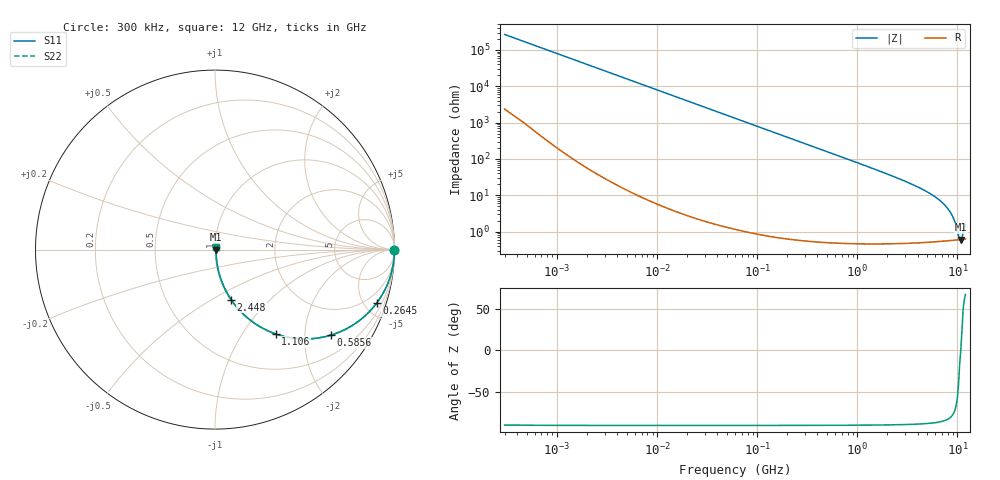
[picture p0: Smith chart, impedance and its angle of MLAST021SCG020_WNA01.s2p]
! MLAST021SCG020_WNA01  S-PARAMETER MODEL  ( General Type )
! Model Generated by TAIYO YUDEN Corporation (http://www.ty-top.com)
! Version 1.0
! TAIYO YUDEN Control No. 220901
! Copyright(c) 2022 TAIYO YUDEN CO.,LTD. All Rights Reserved.
! Product Description (link to TY-COMPAS)
! https://ds.yuden.co.jp/TYCOMPAS/or/detail?pn=MLAST021SCG020BWNA01&u=M
! Products Name : Multilayer Ceramic Capacitors
! Characteristics :
!  Capacitance : 2 pF , Rated Voltage : 25V , TCC : CG / C0G
!  Case Size : 0.25 x 0.125 / 0.0098 x 0.0049 [mm/inch] , Thickness : 0.125 / 0.0049 [mm/inch]
!  (Conditions: Temperature = 25 degC , DC Bias Current/Voltage = 0A / 0V)
! External Node Assignments :
!  1  o---| |---o  2
! GND o---------o GND
! Frequency Range : 0.3MHz  -  12000MHz  [ 401 STEP ]
# MHz S RI R 50
! Freq[MHz].  S11 Real  S11 Imag  S21 Real  S21 Imag  S12 Real  S12 Imag  S22 Real  S22 Imag
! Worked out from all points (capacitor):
!   401 points, 300 kHz to 12 GHz, reference 50 ohm
!   read as one part in series: C = 2 pF near 316.3 kHz
!   lowest |Z| = 606 mohm at 10.79 GHz (marker M1)
!   series resonance near 10.79 GHz, so ESL is about 110 pH
!   S11 on the Smith chart (normalised r, x): 300 kHz: open; 264.5 MHz: 1.01, -6.01; 585.6 MHz: 1.01, -2.71; 1.106 GHz: 1.01, -1.42; 2.448 GHz: 1.01, -0.62; 12 GHz: 1.01, +0.03
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0.3  1 -0.000377  3.48e-06 0.000377  3.48e-06 0.000377  1 -0.000377
1.769972  1 -0.00222  8.37e-06 0.00222  8.37e-06 0.00222  1 -0.00222
10.44266  0.9998 -0.0131  0.000182 0.0131  0.000182 0.0131  0.9998 -0.0131
60  0.9943 -0.075  0.00572 0.075  0.00572 0.075  0.9943 -0.075
129.3602  0.9741 -0.1583  0.0259 0.1583  0.0259 0.1583  0.9741 -0.1583
264.5085  0.8999 -0.2991  0.1001 0.2991  0.1001 0.2991  0.8999 -0.2991
353.9943  0.8339 -0.371  0.1661 0.371  0.1661 0.371  0.8339 -0.371
585.5907  0.6468 -0.4762  0.3532 0.4762  0.3532 0.4762  0.6468 -0.4762
804.7407  0.4916 -0.4975  0.5084 0.4975  0.5084 0.4975  0.4916 -0.4975
1105.905  0.3373 -0.4695  0.6627 0.4695  0.6627 0.4695  0.3373 -0.4695
2088.533  0.1214 -0.3203  0.8786 0.3203  0.8786 0.3203  0.1214 -0.3203
2448.343  0.09 -0.2787  0.91 0.2787  0.91 0.2787  0.09 -0.2787
4623.766  0.0238 -0.1354  0.9762 0.1354  0.9762 0.1354  0.0238 -0.1354
6879.757  0.0098 -0.066  0.9902 0.066  0.9902 0.066  0.0098 -0.066
7854.144  0.00763 -0.0452  0.9924 0.0452  0.9924 0.0452  0.00763 -0.0452
8732.115  0.00656 -0.029  0.9934 0.029  0.9934 0.029  0.00656 -0.029
9454.42  0.00612 -0.0171  0.9939 0.0171  0.9939 0.0171  0.00612 -0.0171
10236.47  0.00597 -0.00524  0.994 0.00524  0.994 0.00524  0.00597 -0.00524
10511.28  0.00599 -0.00185  0.994 0.00185  0.994 0.00185  0.00599 -0.00185
10793.46  0.00602 1.4e-05  0.994 -1.4e-05  0.994 -1.4e-05  0.00602 1.4e-05
11083.22  0.00607 0.00255  0.9939 -0.00255  0.9939 -0.00255  0.00607 0.00255
12000  0.00639 0.0143  0.9936 -0.0143  0.9936 -0.0143  0.00639 0.0143
